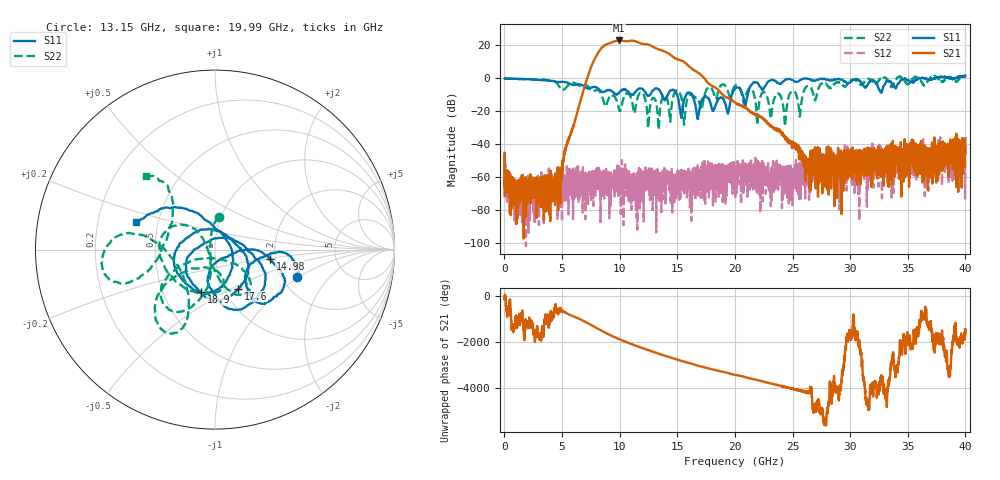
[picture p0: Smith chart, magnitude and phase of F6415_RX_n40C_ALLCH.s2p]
!Keysight Technologies,N5245B,MY52451815,A.15.70.20
!Date: Wednesday, April 17, 2024 15:42:36
!Correction: S33(C  2-Port  )
!S43(C  2-Port  )
!S34(C  2-Port  )
!S44(C  2-Port  )
!S2P File: Measurements: S33, S43, S34, S44:
# Hz S  RI  R 50
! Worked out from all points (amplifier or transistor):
!   4000 points, 10 MHz to 40 GHz, reference 50 ohm
!   highest |S21| = 22.6 dB at 9.94 GHz (marker M1)
!   |S21| within 3 dB of that: 8.67 GHz to 12.67 GHz (4.003 GHz wide, 37.5 % of centre)
!   unconditionally stable (mu >= 1): start of sweep to 32.69 GHz; 33.06 GHz to 34.06 GHz; 34.49 GHz to 35.51 GHz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
!   at 6.67 GHz: K = 829.28, MAG = -8.1 dB, |S12| = -60.1 dB
!   at 20.01 GHz: K = 737.92, MAG = -12.1 dB, |S12| = -54.1 dB
!   at 40 GHz: K = 559.37, MSG = 5.9 dB, |S12| = -48.4 dB
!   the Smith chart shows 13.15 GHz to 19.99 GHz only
!   S11 on the Smith chart (normalised r, x): 13.15 GHz: 2.42, -0.98; 14.98 GHz: 1.87, -0.21; 17.6 GHz: 1.16, -0.54; 18.9 GHz: 0.77, -0.39; 19.99 GHz: 0.37, +0.15
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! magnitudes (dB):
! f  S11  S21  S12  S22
! 10 MHz  -0.4  -71.2  -52.9  -0.6
! 1.47 GHz  -0.7  -70.5  -63.4  -0.7
! 4.55 GHz  -2.4  -58.8  -72.6  -3.2
! 6.68 GHz  -4.2  -11.6  -68.4  -4.8
! 8.2 GHz  -6.9  16.0  -57.9  -7.8
! 9.94 GHz  -9.0  22.6  -68.4  -18.8
! 13.15 GHz  -6.3  17.8  -61.5  -14.8
! 13.34 GHz  -6.8  17.3  -63.4  -27.4
! 14.98 GHz  -10.2  11.2  -61.7  -7.6
! 15.61 GHz  -12.7  9.5  -61.7  -27.2
! 17.6 GHz  -11.9  -2.6  -58.5  -6.4
! 18.9 GHz  -12.0  -9.9  -66.4  -4.0
! 19.99 GHz  -6.6  -14.8  -59.7  -5.0
! 20.01 GHz  -6.4  -15.0  -54.1  -4.8
! 21.94 GHz  -2.9  -22.7  -49.8  -28.0
! 23.8 GHz  -3.4  -31.4  -53.3  -9.6
! 24.34 GHz  -1.4  -35.7  -59.5  -29.3
! 24.91 GHz  -1.1  -39.5  -62.6  -8.1
! 25.62 GHz  -1.5  -45.3  -56.7  -23.2
! 26.67 GHz  -1.5  -46.1  -48.7  -6.9
! 33.34 GHz  -2.2  -65.9  -46.0  -2.5
! 40 GHz  1.3  -36.6  -48.4  0.7
